(* Logix 5000 Rung export; software revision 19.01 *)

TYPE PLX51DF1Input :
STRUCT
   Instance : STRING;
   Status : PLX51DF1Status;
   TransactionRate : DINT;   // The transaction rate is the number of DF1 messages per second that the module is routing
   Temperature : REAL;   // The internal temperature of the module
   DF1RxPacketCount : DINT;   // The number of DF1 packets received by the module
   DF1TxPacketCount : DINT;   // The number of DF1 packets sent by the module
   DF1ChecksumErrors : DINT;   // The number of corrupted DF1 packets received by the module
   PCCCRequests : DINT;   // The number of Ethernet/IP PCCC request sent
   PCCCFailures : DINT;   // The number of failed Ethernet/IP PCCC responses received by the module
   TagReads : DINT;   // The total number of tags reads executed by the module
   TagWrites : DINT;   // The total number of tags writes executed by the module
   TagConnectionFailures : DINT;   // The number of failed class 3 connection attempts
   TagErrors : DINT;   // The number of failed tag access (read/write) requests
END_STRUCT
END_TYPE

TYPE PLX51DF1RMsgRequest :   // Message Request Parameters
STRUCT
   DestinationNode : INT;
   DF1DataFileAddress : STRING;
   Function : PLX51DF1RMsgFunctionType;
   DataType : PLX51DF1RMsgDataType;
   ElementCount : INT;
   RequestData : INT[128];
END_STRUCT
END_TYPE

TYPE PLX51DF1ROutput :   // This parameter is used for the Output Assembly
STRUCT
   RoutingInhibit : BOOL;
END_STRUCT
END_TYPE

TYPE PLX51DF1Status :   // This section reflects the status of the unit
STRUCT
   BridgeMode : BOOL;
   DF1SlaveMode : BOOL;
   ScheduledMode : BOOL;
   UnscheduledMode : BOOL;
   ConfigurationValid : BOOL;
   RoutingInhibited : BOOL;
   Reserved0 : BOOL;
   Reserved1 : BOOL;
   ScheduledTagStatus0 : BOOL;
   ScheduledTagStatus1 : BOOL;
   ScheduledTagStatus2 : BOOL;
   ScheduledTagStatus3 : BOOL;
   ScheduledTagStatus4 : BOOL;
   ScheduledTagStatus5 : BOOL;
   ScheduledTagStatus6 : BOOL;
   ScheduledTagStatus7 : BOOL;
   ScheduledTagStatus8 : BOOL;
   ScheduledTagStatus9 : BOOL;
   ScheduledTagStatus10 : BOOL;
   ScheduledTagStatus11 : BOOL;
   ScheduledTagStatus12 : BOOL;
   ScheduledTagStatus13 : BOOL;
   ScheduledTagStatus14 : BOOL;
   ScheduledTagStatus15 : BOOL;
   ScheduledTagStatus16 : BOOL;
   ScheduledTagStatus17 : BOOL;
   ScheduledTagStatus18 : BOOL;
   ScheduledTagStatus19 : BOOL;
END_STRUCT
END_TYPE

TYPE PLX51DF1RMsgFunctionType :
STRUCT
   PLC5TypedRead : BOOL;
   PLC5TypedWrite : BOOL;
   SLCTypedRead : BOOL;
   SLCTypedWrite : BOOL;
END_STRUCT
END_TYPE

TYPE PLX51DF1RMsgResponse :   // Message Response
STRUCT
   Status : INT;
   ResponseLength : INT;
   ResponseData : INT[128];
END_STRUCT
END_TYPE

TYPE PLX51DF1RMsgDataType :
STRUCT
   BOOLEAN : BOOL;
   INT : BOOL;
   REAL : BOOL;
END_STRUCT
END_TYPE

VAR_GLOBAL   (* controller tags *)
   PLX51DF1ENI:O : AB:ETHERNET_MODULE_DINT_4Bytes:O:0;
   PLX51DF1ENI:I : AB:ETHERNET_MODULE_DINT_136Bytes:I:0;
   PLX51DF1MsgResponse : PLX51DF1RMsgResponse;
   PLX51DF1RMsgRequest : PLX51DF1RMsgRequest := (DestinationNode := 5, DF1DataFileAddress := 'N10:0', Function.PLC5TypedRead := 1, DataType.INT := 1, ElementCount := 16);
   PLX51DF1Input : PLX51DF1Input := (Instance := 'DF1 Router', Status.DF1SlaveMode := 1, Status.ConfigurationValid := 1);
   PLX51DF1MsgTrigger : BOOL;   // Message Trigger
   PLX51DF1Output : PLX51DF1ROutput;
   PLX51DF1Message : MESSAGE;
        MessageParameters(MessageType := CIP Generic, RequestedLength := 360, ConnectedFlag := 2, ConnectionPath := PLX51DF1ENI, ServiceCode := 16#006a, ObjectType := 16#0408, TargetObject := 1, LocalElement := PLX51DF1RMsgRequest, DestinationTag := PLX51DF1MsgResponse)
END_VAR

PROGRAM MainProgram

ROUTINE MainRoutine   (* ladder *)
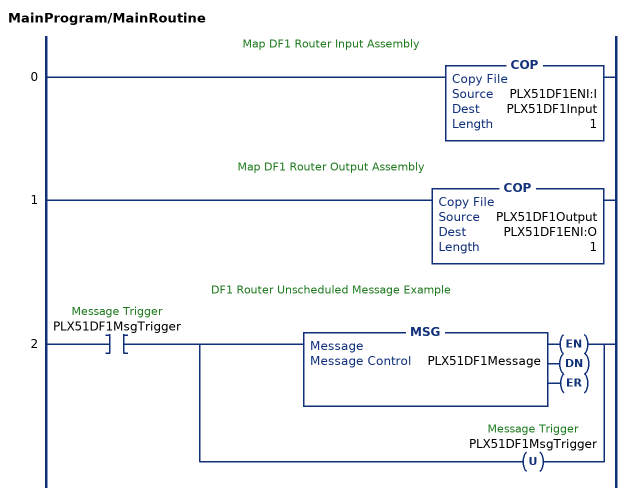
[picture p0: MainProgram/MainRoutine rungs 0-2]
   // Map DF1 Router Input Assembly
   0: COP(PLX51DF1ENI:I,PLX51DF1Input,1);
   // Map DF1 Router Output Assembly
   1: COP(PLX51DF1Output,PLX51DF1ENI:O,1);
   // DF1 Router Unscheduled Message Example
   2: XIC(PLX51DF1MsgTrigger)[MSG(PLX51DF1Message) ,OTU(PLX51DF1MsgTrigger) ];
END_ROUTINE
END_PROGRAM
